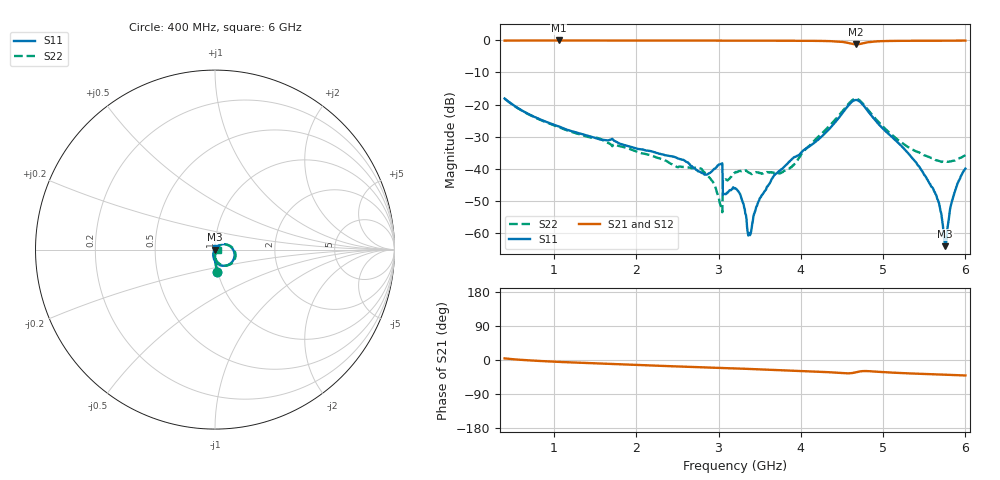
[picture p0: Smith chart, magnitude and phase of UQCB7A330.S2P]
!  Part Number  UQCB7A330	Mounting Orientation: Vertical
!  Description: RF capacitors
!  Application: Coupling, Bypass, Tuning, DC Block
!  Filters, Matching
# GHZ S DB R 50
! Freq  |S11|  S11 Ph  |S21|  S21 Ph  |S12|  S12 Ph  |S22|  S22 Ph
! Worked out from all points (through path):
!   801 points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, 400 MHz to 6 GHz, reference 50 ohm
!   highest |S21| = -0.05 dB at 1.058 GHz (marker M1); lowest = -1.2 dB at 4.67 GHz (marker M2)
!   group delay of S21, straight-line fit = 20.5 ps
!   lowest |S11| = -64.1 dB at 5.755 GHz (marker M3), VSWR 1.00, Z = 50 - j0.0399 ohm
!   |S11| at or under -10 dB: start of sweep to end of sweep
!   |S22| runs from -53.5 to -18.2 dB; largest |S21 - S12| = 0.0012
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0.4  -18.13 -84.2  -0.10 4.2  -0.10 4.2  -18.17 -84.2
1.058  -26.84 -91.3  -0.05 -5.0  -0.05 -5.0  -27.06 -89.9
1.338  -29.20 -92.8  -0.05 -7.6  -0.05 -7.6  -29.47 -89.8
2.269  -35.22 -97.0  -0.07 -15.2  -0.07 -15.2  -36.68 -87.7
2.787  -41.20 -83.6  -0.09 -19.1  -0.09 -19.1  -39.94 -84.2
2.934  -40.35 -54.3  -0.09 -20.3  -0.09 -20.3  -44.16 -101.9
3.018  -38.61 -53.7  -0.10 -21.0  -0.10 -21.0  -50.89 -126.8
3.081  -47.85 -14.3  -0.11 -21.5  -0.11 -21.4  -43.30 -10.0
3.2  -46.03 -22.2  -0.12 -22.2  -0.11 -22.2  -41.21 1.4
3.284  -49.57 -39.7  -0.10 -22.8  -0.10 -22.8  -40.66 -1.8
3.375  -59.99 6.3  -0.10 -23.6  -0.09 -23.6  -41.27 -6.5
3.48  -50.56 63.6  -0.10 -24.5  -0.10 -24.5  -41.11 0.1
3.669  -42.37 71.5  -0.12 -26.1  -0.12 -26.1  -41.31 10.7
3.886  -37.17 62.9  -0.15 -27.8  -0.15 -27.8  -39.53 39.3
4.138  -32.42 50.9  -0.17 -30.0  -0.17 -30.0  -32.02 47.0
4.67  -18.59 -31.7  -1.25 -32.4  -1.25 -32.4  -18.21 -29.7
5.069  -29.22 -106.4  -0.21 -32.8  -0.21 -32.8  -28.57 -89.2
5.622  -47.12 -106.0  -0.14 -37.8  -0.13 -37.8  -37.01 -54.8
5.685  -51.39 -100.7  -0.13 -38.3  -0.13 -38.3  -37.61 -46.0
5.755  -64.11 -39.7  -0.12 -38.8  -0.12 -38.8  -37.79 -34.7
5.86  -48.13 50.0  -0.10 -39.7  -0.10 -39.7  -37.46 -19.0
6  -39.97 47.1  -0.09 -40.9  -0.09 -40.9  -35.75 -2.2
